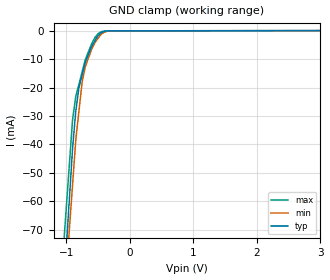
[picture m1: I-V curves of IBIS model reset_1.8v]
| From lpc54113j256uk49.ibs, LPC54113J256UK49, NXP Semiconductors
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[Model] reset_1.8v
Model_type Input
Vinl = 540.000mV
Vinh = 1.44000V
C_comp 1.42000pF 1.40000pF 1.44000pF
[Model spec]
| variable typ   min   max
Vinl  0.540  0.485  0.594
Vinh  1.440  1.296  1.584
| variable typ   min   max
[Voltage Range] 1.80000V 1.62000V 1.98000V
[POWER Clamp Reference] 1.80000V 1.62000V 1.98000V
[GND Clamp Reference] 0.00000V 0.00000V 0.00000V
[Temperature Range]   25   85   -40
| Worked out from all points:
|   GND clamp passes 1 mA (typ) near -0.47 V on its own axis
[GND Clamp]
-1.8V     -359.7mA   -334.7mA   -313.1mA
-900mV    -41.3mA    -54.04mA   -31.22mA
-850mV    -28.3mA    -38.44mA   -23.12mA
-800mV    -20mA      -28.26mA   -18.8mA
-750mV    -15.56mA   -18.07mA   -14.49mA
-700mV    -11.11mA   -12.64mA   -10.17mA
-600mV    -5.518mA   -6.508mA   -4.572mA
-550mV    -3.606mA   -4.224mA   -2.462mA
-450mV    -687uA     -1.224mA   -351.6uA
-350mV    -77.94uA   -170.2uA   -91.49uA
-175mV    -44.4uA    -42.08uA   -49.89uA
3.6V      38.94uA    44.55uA    34.61uA
[POWER Clamp]
-1.8V     0A         0A         0A
3.6V      0A         0A         0A
